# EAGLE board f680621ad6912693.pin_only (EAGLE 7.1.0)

Size 17.78 x 33.02 mm. Coordinates in mm from the lower left corner, seen from the top.
Outline: 0,0 0,33.02 17.78,33.02 17.78,0 0,0
Copper layers (1*2*15*16): Top 0.035mm / dielectric 1.5mm / Route2 0.035mm / dielectric 0.15mm / Route15 0.035mm / dielectric 0.2mm / Bottom 0.035mm
Design rules "SparkFun-4-layer *": minimum track width 6mil, minimum drill 10mil, track to track 6mil, track to pad 6mil, pad to pad 6mil, via to via 6mil, smd to smd 6mil, copper to edge 6mil, drill to drill 8mil, minimum pad ring 12mil, minimum via ring 10mil, stop-mask expansion 4mil, vias tented up to drill 20mil, thermal gap 12mil

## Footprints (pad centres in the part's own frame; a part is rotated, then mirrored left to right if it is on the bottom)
0402-CAP = smd 0.85 x 0.9: 1 -0.58,0; 2 0.58,0
0805-CAP = smd 0.8 x 1.2: 1 -0.9,0; 2 0.9,0
0603-CAP = smd 1.1 x 1: 1 -0.85,0; 2 0.85,0
LED-0603 = smd 1 x 1: A 0,-0.877; C 0,0.877
PTC-1206 = smd 1 x 1.8: 1 -1.4,0; 2 1.4,0
FIDUCIAL-1X2 = smd 1 x 1: 1 0,0
1X12_NO_SILK = drill 1.016 pad 1.88: 1 0,0; 2 2.54,0; 3 5.08,0; 4 7.62,0; 5 10.16,0; 6 12.7,0; 7 15.24,0; 8 17.78,0; 9 20.32,0; 10 22.86,0; 11 25.4,0; 12 27.94,0
USB-AB-MICRO-SMD_V03 = smd 1.4 x 0.4: D+1 2.7,0; D-1 2.7,0.65; GND1 2.7,-1.3; ID1 2.7,-0.65; VBUS1 2.7,1.3 | smd 1.5 x 1.8: SHIELD1 0,3.68; SHIELD3 0,-3.68 | smd 1.5 x 2.5: SHIELD2 0,0 | hole 0.85: 2.2,1.9; 2.2,-1.9
1X02_NO_SILK = drill 1.016 pad 1.88: 1 0,0; 2 2.54,0
2X5-PTH-1.27MM = drill 0.508 pad 1: 1 -2.54,-0.635; 2 -2.54,0.635; 3 -1.27,-0.635; 4 -1.27,0.635; 5 0,-0.635; 6 0,0.635; 7 1.27,-0.635; 8 1.27,0.635; 9 2.54,-0.635; 10 2.54,0.635
0603 = smd 1.1 x 1: 1 -0.85,0; 2 0.85,0
SOT323 = smd 0.7 x 0.7: 1 -0.65,-0.925; 2 0.65,-0.925; 3 0,0.925
SOT23-3 = smd 0.8 x 0.9: 1 -0.95,-1; 2 0.95,-1; 3 0,1.1
0603-RES = smd 1.1 x 1: 1 -0.85,0; 2 0.85,0
TACTILE_SWITCH_SMD_4.6X2.8MM = smd 0.9 x 1: 1 -2.05,-0.8; 2 2.05,-0.8; 3 2.05,0.8; 4 -2.05,0.8
PAD-JUMPER-2-NC_BY_TRACE_NO_SILK = smd 0.635 x 1.27: 1 -0.508,0; 2 0.508,0
TQFP-48 = smd 1.5 x 0.28: 1 -4.25,2.75; 2 -4.25,2.25; 3 -4.25,1.75; 4 -4.25,1.25; 5 -4.25,0.75; 6 -4.25,0.25; 7 -4.25,-0.25; 8 -4.25,-0.75; 9 -4.25,-1.25; 10 -4.25,-1.75; 11 -4.25,-2.25; 12 -4.25,-2.75; 25 4.25,-2.75; 26 4.25,-2.25; 27 4.25,-1.75; 28 4.25,-1.25; 29 4.25,-0.75; 30 4.25,-0.25; 31 4.25,0.25; 32 4.25,0.75; 33 4.25,1.25; 34 4.25,1.75; 35 4.25,2.25; 36 4.25,2.75 | smd 0.28 x 1.5: 13 -2.75,-4.25; 14 -2.25,-4.25; 15 -1.75,-4.25; 16 -1.25,-4.25; 17 -0.75,-4.25; 18 -0.25,-4.25; 19 0.25,-4.25; 20 0.75,-4.25; 21 1.25,-4.25; 22 1.75,-4.25; 23 2.25,-4.25; 24 2.75,-4.25; 37 2.75,4.25; 38 2.25,4.25; 39 1.75,4.25; 40 1.25,4.25; 41 0.75,4.25; 42 0.25,4.25; 43 -0.25,4.25; 44 -0.75,4.25; 45 -1.25,4.25; 46 -1.75,4.25; 47 -2.25,4.25; 48 -2.75,4.25
SOT23-5 = smd 0.55 x 1.2: 1 -0.95,-1.3; 2 0,-1.3; 3 0.95,-1.3; 4 0.95,1.3; 5 -0.95,1.3
CRYSTAL-SMD-3.2X1.5MM = smd 1 x 1.8: P$1 -1.25,0; P$2 1.25,0

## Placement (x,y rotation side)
C1  0.1uF  [0402-CAP]  4.39,18.54 180 top
C2  0.1uF  [0402-CAP]  3.17,12.19 270 top
C3  0.1uF  [0402-CAP]  8.89,7.37 270 top
C4  0.1uF  [0402-CAP]  14.61,13.21 90 top
C5  15pF  [0402-CAP]  3.81,9.53 0 top
C6  15pF  [0402-CAP]  7.62,7.37 270 top
C7  1.0uF  [0805-CAP]  5.08,21.21 270 top
C8  2.2uF  [0603-CAP]  10.16,22.23 90 top
D1  GREEN  [LED-0603]  3.81,1.91 0 top
D2  RED  [LED-0603]  1.91,30.99 270 top
D3  BLUE  [LED-0603]  15.88,30.99 90 top
D4  Yellow  [LED-0603]  13.97,1.91 0 top
F1  500mA  [PTC-1206]  13.97,26.67 270 top
FID1  FIDUCIAL1X2  [FIDUCIAL-1X2]  15.24,2.54 0 top
FID2  FIDUCIAL1X2  [FIDUCIAL-1X2]  3.68,28.96 0 top
FRAME1  FRAME-LETTER  [CREATIVE_COMMONS]  not placed on the board
JP1  [1X12_NO_SILK]  1.27,1.27 90 top
JP2  [1X12_NO_SILK]  16.51,29.21 270 top
JP3  [USB-AB-MICRO-SMD_V03]  8.89,31.11 270 top
JP4  [1X02_NO_SILK]  13.59,17.91 90 top
JP5  CORTEX_DEBUGPTH  [2X5-PTH-1.27MM]  8.89,4.67 0 top
L1  FB - 30Ohm  [0603]  11.43,7.37 180 top
LOGO1  SFE_LOGO_FLAME.1_INCH  [SFE_LOGO_FLAME_.1]  10.54,18.92 0 top
LOGO2  OSHW-LOGOS  [OSHW-LOGO-S]  5.33,17.63 90 bottom
LOGO3  SFE_LOGO_NAME_FLAME.1_INCH  [SFE_LOGO_NAME_FLAME_.1]  7.21,5.94 90 bottom
Q1  2N7002PW  [SOT323]  13.97,22.86 0 top
Q2  2.5A/30V  [SOT23-3]  11.18,25.4 270 top
R1  10K  [0603-RES]  13.97,6.35 90 top
R2  330  [0603-RES]  1.91,32.26 0 top
R3  330  [0603-RES]  15.88,32.26 180 top
R4  100k  [0603-RES]  6.35,25.4 270 top
R5  330  [0603-RES]  7.62,25.4 90 top
R6  330  [0603-RES]  5.08,1.91 90 top
R7  47K  [0603-RES]  8.89,25.4 270 top
R8  330  [0603-RES]  12.7,1.91 90 top
S1  RESET  [TACTILE_SWITCH_SMD_4.6X2.8MM]  8.89,1.4 180 top
SJ1  PWR-LED  [PAD-JUMPER-2-NC_BY_TRACE_NO_SILK]  1.91,31.62 0 bottom
U1  ATSAMD21G-A  [TQFP-48]  8.89,13.72 90 top
U2  3.3V  [SOT23-5]  7.62,21.21 180 top
U3  74AHC1G125  [SOT23-5]  3.81,25.4 180 top
Y1  32.768kHz  [CRYSTAL-SMD-3.2X1.5MM]  4.95,7.37 180 top

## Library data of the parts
C1-C4 = SparkFun-Capacitors; PROD_ID: CAP-12416
C5 C6 = samd21-temp; PROD_ID: CAP-13063
C7 = SparkFun-Capacitors; PROD_ID: CAP-11625
C8 = SparkFun-Capacitors; PROD_ID: CAP-07888
D1 = SparkFun-LED; PROD_ID: DIO-00821
D2 = SparkFun-LED; PROD_ID: DIO-00819
D3 = SparkFun-LED; PROD_ID: DIO-08575
D4 = SparkFun-LED; PROD_ID: DIO-09003
F1 = SparkFun-PowerIC; PROD_ID: RES-11150
FID1 FID2 FRAME1 LOGO1-LOGO3 = SparkFun-Aesthetics
JP1 JP2 JP4 = SparkFun-Connectors
JP3 = SparkFun-Connectors; PROD_ID: CONN-11794
JP5 = samd21-temp
L1 = SparkFun-Passives; PROD_ID: RES-07859
Q1 = SparkFun-DiscreteSemi; PROD_ID: TRANS-11151
Q2 = SparkFun-DiscreteSemi; PROD_ID: TRANS-11308
R1 = SparkFun-Resistors; PROD_ID: RES-00824
R2 R3 R5 R6 R8 = SparkFun-Resistors; PROD_ID: RES-00818
R4 = SparkFun-Resistors; PROD_ID: RES-07828
R7 = SparkFun-Resistors; PROD_ID: RES-07871
S1 = samd21-temp; PROD_ID: SWCH-13065
SJ1 = SparkFun-Passives
U1 = samd21-temp; PROD_ID: IC-13064
U2 = SparkFun-PowerIC; PROD_ID: VREG-12457
U3 = SparkFun-DigitalIC; PROD_ID: IC-11920
Y1 = samd21-temp; PROD_ID: XTAL-13062

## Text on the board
Bottom: v10
tPlace: PWR | 13 | 1 | VIN | GND | 2 | A3 | 3 | A2 | 4 | 5 | A0 | 6 | 13 | 7 | 12 | 8 | 11 | TX | RX | 9 | 10
bPlace: PWR / LED | 1/TX | VIN | 0/RX | GND | !RST | AREF | SAMD21G Mini / Breakout | GND | VCC | SCL | 2 | A3 | SDA | 3 | A2 | 4 | A1 | 5 | A0 | 6 | 13 | 7 | 12 | 8 | 11 | 9 | 10
Measures: Units in inches
tDocu: This is a 4-layer board! | Jim Lindblom

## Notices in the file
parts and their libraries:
SparkFun-Connectors: Licensing: Creative Commons ShareAlike 4.0 International - https://creativecommons.org/licenses/by-sa/4.0
SparkFun-Aesthetics: Released under the Creative Commons Attribution Share-Alike 4.0 License
SparkFun-Aesthetics: https://creativecommons.org/licenses/by-sa/4.0
